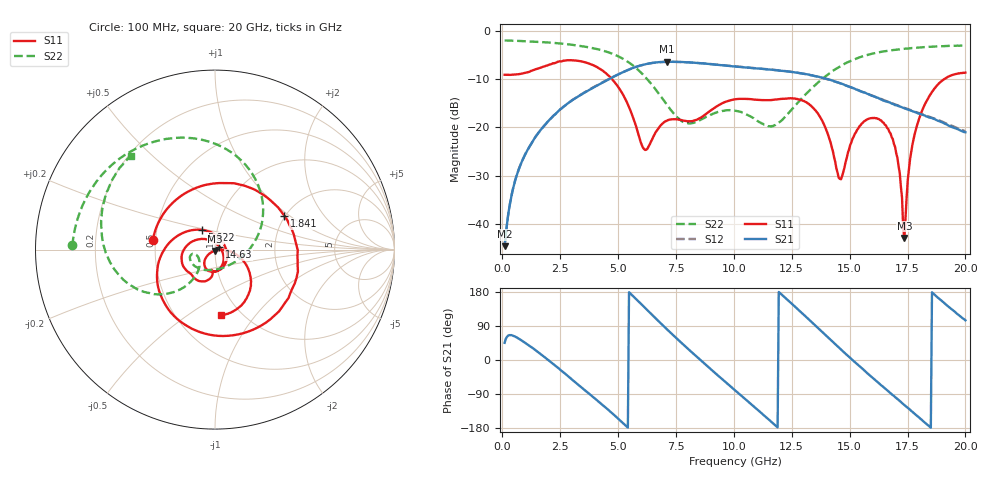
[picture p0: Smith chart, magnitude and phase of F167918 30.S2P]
!  2-Port S-parameters saved by WinCal
! VAR MeasName=S-Parameters (CALIBRATED_DATA) read from VNA (N5242A)
! VAR MeasDate=2016-11-22 10:26:11
! VAR NAME=F167918 30
! VAR FILENAME=F167918 30.S2P
! VAR DATE=2016-11-22 10:26:11
! VAR PHYS_PORTS=1,2
# Hz S DB R 50
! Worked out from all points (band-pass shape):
!   401 points, 100 MHz to 20 GHz, reference 50 ohm
!   highest |S21| = -6.41 dB at 7.115 GHz (marker M1); lowest = -44.6 dB at 100 MHz (marker M2)
!   |S21| within 3 dB of the highest: 4.854 GHz to 13.54 GHz (8.685 GHz wide, 94.4 % of centre)
!   lowest |S11| = -43.0 dB at 17.36 GHz (marker M3), VSWR 1.01, Z = 50.1 - j0.7 ohm
!   |S11| at or under -10 dB: 4.737 GHz to 19.09 GHz (14.35 GHz wide, 120 % of centre)
!   |S22| runs from -19.9 to -2.0 dB; largest |S21 - S12| = 0.0042
!   S11 on the Smith chart (normalised r, x): 100 MHz: 0.48, +0.06; 1.841 GHz: 1.97, +0.91; 5.622 GHz: 0.85, +0.19; 14.63 GHz: 1.05, +0.03; 20 GHz: 0.81, -0.69
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1e8  -9.12 171.0  -44.65 45.3  -44.52 45.3  -2.00 178.3
6.97e8  -9.00 119.0  -28.91 56.9  -28.88 56.6  -2.09 168.7
1.84125e9  -7.35 26.1  -19.49 6.8  -19.50 6.7  -2.37 150.1
2.53775e9  -6.34 -26.4  -16.17 -27.6  -16.16 -27.4  -2.64 137.9
3.43325e9  -6.36 -87.6  -13.15 -73.1  -13.09 -72.9  -3.19 120.4
4.478e9  -8.81 -152.8  -10.36 -126.4  -10.30 -126.7  -4.30 95.1
5.62225e9  -17.62 123.6  -7.74 170.1  -7.74 169.7  -7.12 57.9
6.1695e9  -24.70 30.3  -6.94 137.4  -6.95 137.2  -9.55 36.5
6.7665e9  -20.05 -56.6  -6.49 101.4  -6.51 101.4  -13.08 10.2
7.11475e9  -18.59 -78.8  -6.41 80.9  -6.43 81.0  -15.35 -7.5
8.50775e9  -18.19 -96.1  -6.71 2.5  -6.68 2.6  -18.57 -102.3
1.005e10  -14.20 -115.4  -7.38 -79.9  -7.37 -79.8  -16.58 -160.0
1.17415e10  -14.29 -139.0  -8.12 -169.8  -8.09 -169.9  -19.58 -148.5
1.338325e10  -15.80 174.1  -9.23 98.6  -9.24 98.8  -11.83 -128.6
1.4627e10  -30.79 30.2  -10.94 27.8  -10.93 27.9  -7.26 -145.7
1.5622e10  -18.77 -80.6  -12.78 -26.8  -12.78 -26.4  -5.21 -164.1
1.67165e10  -20.95 -131.0  -14.82 -84.9  -14.82 -84.4  -4.11 176.8
1.706475e10  -26.31 -142.4  -15.52 -102.8  -15.43 -102.6  -3.88 171.4
1.736325e10  -42.95 -78.6  -16.06 -118.7  -15.98 -118.0  -3.73 167.1
1.77115e10  -23.61 -2.5  -16.67 -136.7  -16.56 -136.4  -3.57 162.0
1.815925e10  -16.20 -19.0  -17.43 -160.3  -17.33 -159.9  -3.41 155.7
2e10  -8.67 -84.4  -21.03 104.7  -20.82 104.8  -3.08 131.8
